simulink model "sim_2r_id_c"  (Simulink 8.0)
settings: Solver=ode45  StartTime=0.0  StopTime=5  RelTol=1e-3
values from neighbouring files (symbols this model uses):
  m = 1    [mechanical_system.m]
  s = Lv/norm(Lv)    [pkm1.m]
undefined symbols (not defined in the file or in its folder): deg, kg, mN, N, rad
libraries: mblibv1 x12

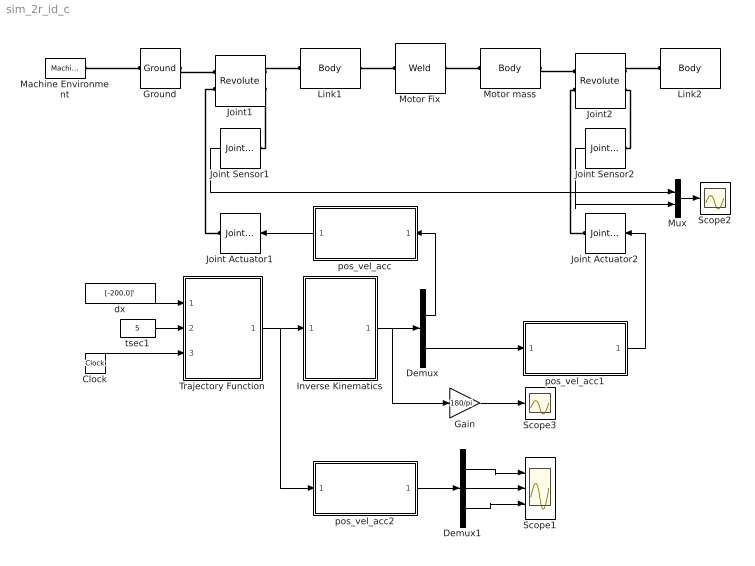
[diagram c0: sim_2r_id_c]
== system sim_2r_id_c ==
  Clock : Clock
  Demux : Demux  Outputs=2
  Demux1 : Demux  Outputs=3
  Gain : Gain  Gain=180/pi
  Ground : mblibv1/Bodies/Ground  UpdateFromCAD=off  LeftPortType=env  RightPortType=workingframe  PhysicalDomain=Mechanical  DialogClass=GroundBlock  CoordPosition=[0 0 0]  CoordPositionUnits=m  StateVectorMgrId=-1  MachineId=[0 0]  ShowEnvPort=on
  Inverse Kinematics : MATLAB Function  TreatAsAtomicUnit=on
  Joint Actuator1 : mblibv1/Sensors &  Actuators/Joint Actuator  UpdateFromCAD=off  PhysicalDomain=Mechanical  PortType=blob  ActuationStyle=Motion  AngleUnits=rad  ArcVelocityUnits=rad/s  ArcAccelerationUnits=rad/s^2  CoordPositionUnits=m  VelocityUnits=m/s  AccelerationUnits=m/s^2  ForceUnits=N  TorqueUnits=N*m  ActiveIO=on  Width=3  DialogClass=MechanicalActuatorBlock  Primitive=R1  ReferenceFrame=Absolute (World)
  Joint Actuator2 : mblibv1/Sensors &  Actuators/Joint Actuator  UpdateFromCAD=off  PhysicalDomain=Mechanical  PortType=blob  ActuationStyle=Motion  AngleUnits=rad  ArcVelocityUnits=rad/s  ArcAccelerationUnits=rad/s^2  CoordPositionUnits=m  VelocityUnits=m/s  AccelerationUnits=m/s^2  ForceUnits=N  TorqueUnits=N*m  ActiveIO=on  Width=3  DialogClass=MechanicalActuatorBlock  Primitive=R1  ReferenceFrame=Absolute (World)
  Joint Sensor1 : mblibv1/Sensors &  Actuators/Joint Sensor  UpdateFromCAD=off  PhysicalDomain=Mechanical  PortType=blob  Muxed=on  Pose=off  Angle=off  AngleUnits=deg  ArcVelocity=off  ArcVelocityUnits=deg/s  ArcAcceleration=off  ArcAccelerationUnits=deg/s^2  CoordPosition=on  CoordPositionUnits=m  Velocity=off  VelocityUnits=m/s  Acceleration=off  AccelerationUnits=m/s^2  Quaternion=on  QuaternionDT=off  QuaternionDDT=off  QuaternionUnits=off  OutputVector=[1]  ActiveIO=on  Width=1  DialogClass=MechanicalSensorBlock  Primitive=R1  Force=off  ForceUnits=N  Torque=on  TorqueUnits=mN*m  ReferenceFrame=Absolute (World)  ReactionSensedSide=Base  ReactionReferenceFrame=Absolute (World)  ReactionForce=off  ReactionForceUnits=N  ReactionMoment=off  ReactionMomentUnits=N*m
  Joint Sensor2 : mblibv1/Sensors &  Actuators/Joint Sensor  UpdateFromCAD=off  PhysicalDomain=Mechanical  PortType=blob  Muxed=on  Pose=off  Angle=off  AngleUnits=deg  ArcVelocity=off  ArcVelocityUnits=deg/s  ArcAcceleration=off  ArcAccelerationUnits=deg/s^2  CoordPosition=on  CoordPositionUnits=m  Velocity=off  VelocityUnits=m/s  Acceleration=off  AccelerationUnits=m/s^2  Quaternion=on  QuaternionDT=off  QuaternionDDT=off  QuaternionUnits=off  OutputVector=[1]  ActiveIO=on  Width=1  DialogClass=MechanicalSensorBlock  Primitive=R1  Force=off  ForceUnits=N  Torque=on  TorqueUnits=mN*m  ReferenceFrame=Absolute (World)  ReactionSensedSide=Base  ReactionReferenceFrame=Absolute (World)  ReactionForce=off  ReactionForceUnits=N  ReactionMoment=off  ReactionMomentUnits=N*m
  Joint1 : mblibv1/Joints/Revolute  LConnTagsString=__newl0|SA1  RConnTagsString=__newr0|SA1  UpdateFromCAD=off  NumSAPorts=2  CutJoint=off  MarkAsCut=off  Primitives=prismatic  PrimitiveProps=R1$World$[0 0 1]$revolute  DialogClass=JointBlock  R1Axis=[0 0 1]
  Joint2 : mblibv1/Joints/Revolute  LConnTagsString=__newl0|SA1  RConnTagsString=__newr0|SA1  UpdateFromCAD=off  NumSAPorts=2  CutJoint=off  MarkAsCut=off  Primitives=prismatic  PrimitiveProps=R1$World$[0 0 1]$revolute  DialogClass=JointBlock  R1Axis=[0 0 1]
  Link1 : mblibv1/Bodies/Body  LConnTagsString=CS1  RConnTagsString=CS2  UpdateFromCAD=off  DialogClass=MechanicalBodyBlock  Mass=0.071  MassUnits=kg  InertiaUnits=kg*m^2  Inertia=[0 0 0; 0 0 0; 0 0 0.000089395]  Shape=Cylinder  ShapeDims=[1 1]  ShapeUnits=m  ShapeUse=false  Density=1  DensityUnits=kg/m^3  DensityUse=false  GraphicsMode=MACHINE_DEFAULT  BodyColorSelMode=MACHINE_DEFAULT  BodyColor=[1 0 0]  AttachedToCS=CG  CG=Left$CG$[0.0373 0 0]$CS1$CS1$m$[0 0 0]$Euler X-Y-Z$deg$WORLD$false$none  WorkingFrames=Left$CS1$[0 0 0]$World$World$m$[0 0 0]$Euler X-Y-Z$deg$WORLD$true$none#Right$CS2$[0.1 0 0]$World$World$m$[0 0 0]$Euler X-Y-Z$deg$WORLD$true$none  CGPos=[0.0373 0 0]  CGRot=[0 0 0]  CS0Pos=[]  CS0Rot=[]  CS1Pos=[0 0 0]  CS1Rot=[0 0 0]  CS2Pos=[0.1 0 0]  CS2Rot=[0 0 0]  CS3Pos=[]  CS3Rot=[]  CS4Pos=[]  CS4Rot=[]  CS5Pos=[]  CS5Rot=[]  CS6Pos=[]  CS6Rot=[]  CS7Pos=[]  CS7Rot=[]  CS8Pos=[]  CS8Rot=[]  CS9Pos=[]  CS9Rot=[]  CS10Pos=[]  CS10Rot=[]  CS11Pos=[]  CS11Rot=[]  CS12Pos=[]  CS12Rot=[]  CS13Pos=[]  CS13Rot=[]  CS14Pos=[]  CS14Rot=[]  CS15Pos=[]  CS15Rot=[]  CS16Pos=[]  CS16Rot=[]  CS17Pos=[]  CS17Rot=[]  CS18Pos=[]  CS18Rot=[]  CS19Pos=[]  CS19Rot=[]  CS20Pos=[]  CS20Rot=[]
  Link2 : mblibv1/Bodies/Body  LConnTagsString=CS1  UpdateFromCAD=off  DialogClass=MechanicalBodyBlock  Mass=0.1  MassUnits=kg  InertiaUnits=kg*m^2  Inertia=[0 0 0; 0 0 0; 0 0 0.000109864]  Shape=Cylinder  ShapeDims=[1 1]  ShapeUnits=m  ShapeUse=false  Density=1  DensityUnits=kg/m^3  DensityUse=false  GraphicsMode=MACHINE_DEFAULT  BodyColorSelMode=MACHINE_DEFAULT  BodyColor=[1 0 0]  AttachedToCS=CG  CG=Left$CG$[0.04168 0 0]$CS1$CS1$m$[0 0 0]$Euler X-Y-Z$deg$WORLD$false$none  WorkingFrames=Left$CS1$[0.1 0 0]$World$World$m$[0 0 0]$Euler X-Y-Z$deg$WORLD$true$none#Right$CS2$[0.2 0 0]$World$World$m$[0 0 0]$Euler X-Y-Z$deg$WORLD$false$none  CGPos=[0.04168 0 0]  CGRot=[0 0 0]  CS0Pos=[]  CS0Rot=[]  CS1Pos=[0.1 0 0]  CS1Rot=[0 0 0]  CS2Pos=[0.2 0 0]  CS2Rot=[0 0 0]  CS3Pos=[]  CS3Rot=[]  CS4Pos=[]  CS4Rot=[]  CS5Pos=[]  CS5Rot=[]  CS6Pos=[]  CS6Rot=[]  CS7Pos=[]  CS7Rot=[]  CS8Pos=[]  CS8Rot=[]  CS9Pos=[]  CS9Rot=[]  CS10Pos=[]  CS10Rot=[]  CS11Pos=[]  CS11Rot=[]  CS12Pos=[]  CS12Rot=[]  CS13Pos=[]  CS13Rot=[]  CS14Pos=[]  CS14Rot=[]  CS15Pos=[]  CS15Rot=[]  CS16Pos=[]  CS16Rot=[]  CS17Pos=[]  CS17Rot=[]  CS18Pos=[]  CS18Rot=[]  CS19Pos=[]  CS19Rot=[]  CS20Pos=[]  CS20Rot=[]
  Machine Environment : mblibv1/Bodies/Machine Environment  PortType=env  PhysicalDomain=Mechanical  DialogTemplateClass=MECH.MachineEnvironment  SyncWhenCopied=off  Gravity=[0 -9.81 0]  GravityUnits=m/s^2  GravityAsSignal=off  Dimensionality=Auto-detect  AnalysisType=Forward dynamics  LinearAssemblyTolerance=1e-3  LinearAssemblyToleranceUnits=m  AngularAssemblyTolerance=1e-3  AngularAssemblyToleranceUnits=rad  ConstraintSolverType=Stabilizing  ConstraintRelTolerance=1e-4  ConstraintAbsTolerance=1e-4  UseRobustSingularityHandling=off  RedundancyAnalysisToleranceType=Automatically select tolerance  RedundancyAnalysisTolerance=1e-14  StatePerturbationType=Fixed  PerturbationSize=1e-5  VisualizeMachine=on  BodyVisualizationType=Use model default body geometries  BodyColorSelMode=Use model default  DefaultBodyColor=[1 0 0]
  Motor Fix : mblibv1/Joints/Weld  LConnTagsString=__newl0  RConnTagsString=__newr0  UpdateFromCAD=off  NumSAPorts=0  CutJoint=off  MarkAsCut=off  Primitives=weld  PrimitiveProps=W$WORLD$[0 0 0]$weld  DialogClass=JointBlock  WAxis=[0 0 0]
  Motor mass : mblibv1/Bodies/Body  LConnTagsString=CS1  RConnTagsString=CS2  UpdateFromCAD=off  DialogClass=MechanicalBodyBlock  Mass=0.292  MassUnits=kg  InertiaUnits=kg*m^2  Inertia=[0 0 0; 0 0 0; 0 0 0]  Shape=Cylinder  ShapeDims=[1 1]  ShapeUnits=m  ShapeUse=false  Density=1  DensityUnits=kg/m^3  DensityUse=false  GraphicsMode=MACHINE_DEFAULT  BodyColorSelMode=MACHINE_DEFAULT  BodyColor=[1 0 0]  AttachedToCS=CG  CG=Left$CG$[0.1 0 0]$WORLD$WORLD$m$[0 0 0]$Euler X-Y-Z$deg$WORLD$false$none  WorkingFrames=Left$CS1$[0.1 0 0]$World$World$m$[0 0 0]$Euler X-Y-Z$deg$WORLD$true$none#Right$CS2$[0.1 0 0]$World$World$m$[0 0 0]$Euler X-Y-Z$deg$WORLD$true$none  CGPos=[0.1 0 0]  CGRot=[0 0 0]  CS0Pos=[]  CS0Rot=[]  CS1Pos=[0.1 0 0]  CS1Rot=[0 0 0]  CS2Pos=[0.1 0 0]  CS2Rot=[0 0 0]  CS3Pos=[]  CS3Rot=[]  CS4Pos=[]  CS4Rot=[]  CS5Pos=[]  CS5Rot=[]  CS6Pos=[]  CS6Rot=[]  CS7Pos=[]  CS7Rot=[]  CS8Pos=[]  CS8Rot=[]  CS9Pos=[]  CS9Rot=[]  CS10Pos=[]  CS10Rot=[]  CS11Pos=[]  CS11Rot=[]  CS12Pos=[]  CS12Rot=[]  CS13Pos=[]  CS13Rot=[]  CS14Pos=[]  CS14Rot=[]  CS15Pos=[]  CS15Rot=[]  CS16Pos=[]  CS16Rot=[]  CS17Pos=[]  CS17Rot=[]  CS18Pos=[]  CS18Rot=[]  CS19Pos=[]  CS19Rot=[]  CS20Pos=[]  CS20Rot=[]
  Mux : Mux  Inputs=2
  Scope1 : Scope  NumInputPorts=3
  Scope2 : Scope
  Scope3 : Scope
  Trajectory Function : MATLAB Function  TreatAsAtomicUnit=on
  dx : Constant  Value=[-200,0]'  SampleTime=-1
  pos_vel_acc : Subsystem
  pos_vel_acc1 : Subsystem
  pos_vel_acc2 : Subsystem
  tsec1 : Constant  Value=5  SampleTime=-1
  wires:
  Joint Sensor1/1 -> Mux/1
  Joint Sensor2/1 -> Mux/2
  pos_vel_acc1/1(Motion2) -> Joint Actuator2/1
  Demux/1 -> pos_vel_acc/1(In1)
  Demux/2 -> pos_vel_acc1/1(In1)
  pos_vel_acc/1(Motion1) -> Joint Actuator1/1
  dx/1 -> Trajectory Function/1(dx)
  tsec1/1 -> Trajectory Function/2(tsec)
  Trajectory Function/1(xd) -> Inverse Kinematics/1(xd), pos_vel_acc2/1(In1)
  Clock/1 -> Trajectory Function/3(tout)
  Inverse Kinematics/1(thd) -> Gain/1, Demux/1
  Demux1/1 -> Scope1/1
  Demux1/2 -> Scope1/2
  Demux1/3 -> Scope1/3
  pos_vel_acc2/1(Motion2) -> Demux1/1
  Mux/1 -> Scope2/1
  Gain/1 -> Scope3/1
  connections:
  Machine Environment/RConn1 -- Ground/LConn1
  Joint1/RConn1 -- Link1/LConn1
  Ground/RConn1 -- Joint1/LConn1
  Link1/RConn1 -- Motor Fix/LConn1
  Motor Fix/RConn1 -- Motor mass/LConn1
  Motor mass/RConn1 -- Joint2/LConn1
  Joint2/RConn1 -- Link2/LConn1
  Joint1/RConn2 -- Joint Sensor1/LConn1
  Joint2/RConn2 -- Joint Sensor2/LConn1
  Joint1/LConn2 -- Joint Actuator1/RConn1
  Joint2/LConn2 -- Joint Actuator2/RConn1

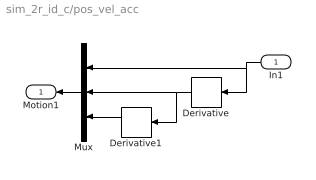
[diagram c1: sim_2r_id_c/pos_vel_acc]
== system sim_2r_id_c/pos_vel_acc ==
  In1 : Inport
  Derivative : Derivative
  Derivative1 : Derivative
  Mux : Mux  Inputs=3
  Motion1 : Outport
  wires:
  Derivative/1 -> Mux/2, Derivative1/1
  Derivative1/1 -> Mux/3
  In1/1 -> Mux/1, Derivative/1
  Mux/1 -> Motion1/1

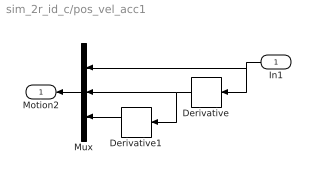
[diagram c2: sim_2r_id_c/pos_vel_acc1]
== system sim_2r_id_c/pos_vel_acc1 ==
  In1 : Inport
  Derivative : Derivative
  Derivative1 : Derivative
  Mux : Mux  Inputs=3
  Motion2 : Outport
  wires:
  Derivative/1 -> Mux/2, Derivative1/1
  Derivative1/1 -> Mux/3
  In1/1 -> Mux/1, Derivative/1
  Mux/1 -> Motion2/1

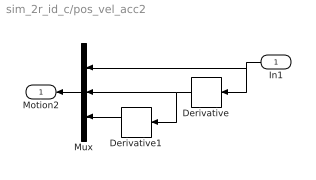
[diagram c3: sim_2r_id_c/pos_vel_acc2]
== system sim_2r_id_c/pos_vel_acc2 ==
  In1 : Inport
  Derivative : Derivative
  Derivative1 : Derivative
  Mux : Mux  Inputs=3
  Motion2 : Outport
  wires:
  Derivative/1 -> Mux/2, Derivative1/1
  Derivative1/1 -> Mux/3
  In1/1 -> Mux/1, Derivative/1
  Mux/1 -> Motion2/1

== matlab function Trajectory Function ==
function xd = fcn(dx, tsec, tout)

MAX_CH=2;       % Two Actuators %
a1=100; a2=100;

% Initializing Variables %
%if isempty(xd_p), xd_p=zeros(MAX_CH,1); end
xd=zeros(MAX_CH,1);
x0=[a1,a2]';

%tout=index*dt;

    [c] = coeff_3rd(x0, zeros(MAX_CH,1), x0+dx, zeros(MAX_CH,1), tsec);
    for ch=1:MAX_CH
        xd(ch,1)=c(ch,1)+c(ch,2)*tout+c(ch,3)*tout^2+c(ch,4)*tout^3;    
    end

function [c] = coeff_3rd(sp, sv, ep, ev, tsec)
MAX_CH=2;
c=zeros(MAX_CH,4);
for ch=1:MAX_CH
    c(ch,1)=sp(ch,1);
    c(ch,2)=sv(ch,1);
    c(ch,3)=(3.0*(ep(ch,1)-sp(ch,1))-(2.0*sv(ch,1)+ev(ch,1))*tsec)/(tsec*tsec);
    c(ch,4)=(-2.0*(ep(ch,1)-sp(ch,1))+(sv(ch,1)+ev(ch,1))*tsec)/(tsec*tsec*tsec);
end

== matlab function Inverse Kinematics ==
function thd   = fcn(xd)

persistent index thd_p

% Initializing Variables %
if isempty(index), index=0; end
if isempty(thd_p), thd_p=(pi/180)*[0,90]'; end

w_index=1;  % In workspace %
a1=100; a2=100;

% (1) Calculate th2 %
px=xd(1,1); py=xd(2,1);
kapha=(px^2+py^2-a1^2-a2^2)/(2*a1*a2);
if abs(kapha)>1
    w_index=-1;  % Out of Workspace %
    kapha=1;
end
th2=+acos(kapha); % Elbow Down %
%th2=-acos(kapha); % Elbow Up %
 
% (2) Calculate th1 %
delta=a1^2+a2^2+2*a1*a2*cos(th2);
cth1=(px*(a1+a2*cos(th2))+py*a2*sin(th2))/delta;
sth1=(-px*a2*sin(th2)+py*(a1+a2*cos(th2)))/delta;
th1=atan2(sth1, cth1);
if th1<0, th1=th1+2*pi; end % 0<th<360 %

% (3) Check Joint Limits %
if th1<0 || th1>pi, w_index=-1; end
if th2<pi/6 || th2>5*pi/6, w_index=-1; end

% Result %
if w_index==1
    thd=[th1, th2]';
else
    thd=thd_p;
end

% Save the current value %
thd_p=thd;
